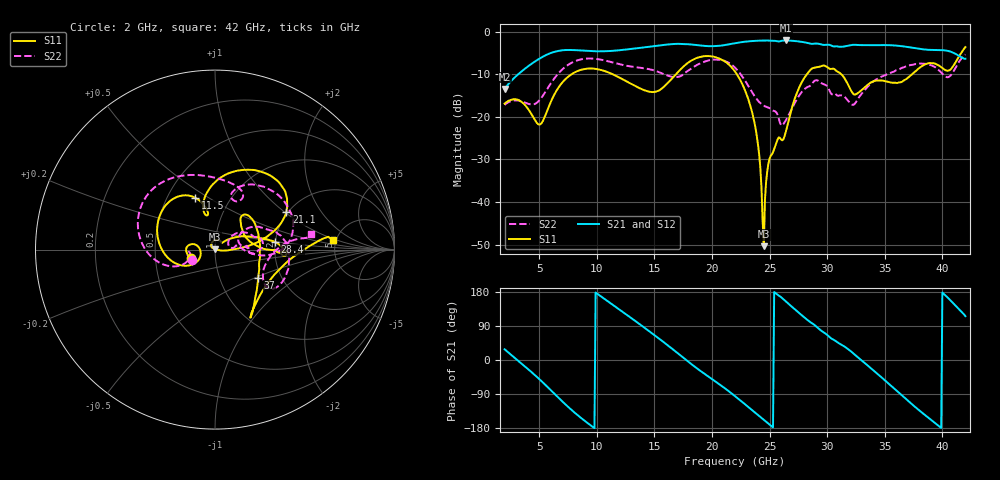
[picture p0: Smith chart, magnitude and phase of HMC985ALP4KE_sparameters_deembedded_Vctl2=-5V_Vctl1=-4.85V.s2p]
!s2p File: Measurements: S11, S21, S12, S22
# GHz S dB R 50.0
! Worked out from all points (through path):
!   401 points, 2 GHz to 42 GHz, reference 50 ohm
!   highest |S21| = -2.06 dB at 26.4 GHz (marker M1); lowest = -13.4 dB at 2 GHz (marker M2)
!   lowest |S11| = -50.4 dB at 24.5 GHz (marker M3), VSWR 1.01, Z = 49.8 + j0.261 ohm
!   |S11| at or under -10 dB: start of sweep to 7.809 GHz; 22.16 GHz to 28.24 GHz (6.081 GHz wide, 24.1 % of centre); 31.22 GHz to 37.36 GHz (6.143 GHz wide, 17.9 % of centre)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
!   |S22| runs from -22.0 to -5.4 dB; largest |S21 - S12| = 0.00096
!   S11 on the Smith chart (normalised r, x): 2 GHz: 0.76, -0.07; 11.5 GHz: 0.68, +0.44; 21.1 GHz: 1.96, +1.02; 28.4 GHz: 1.99, +0.19; 37 GHz: 1.52, -0.52; 42 GHz: 4.71, +0.87
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2  -16.88 -161.7  -13.43 28.3  -13.44 28.3  -17.18 -155.6
5  -21.81 -172.3  -6.37 -50.1  -6.38 -50.1  -16.18 -159.7
6.3  -14.84 -150.2  -4.76 -88.3  -4.76 -88.3  -11.03 -161.5
8.7  -8.91 150.4  -4.44 -154.5  -4.44 -154.5  -6.47 151.4
11.5  -10.16 111.2  -4.47 143.2  -4.48 143.3  -7.31 105.2
13.6  -13.11 101.2  -3.86 97.3  -3.86 97.3  -8.41 75.8
15.4  -13.82 105.8  -3.26 56.6  -3.26 56.6  -9.50 62.2
17.9  -7.34 80.4  -2.95 -3.3  -2.95 -3.3  -9.21 72.2
21.1  -6.97 27.7  -3.15 -74.2  -3.15 -74.1  -6.87 16.3
22  -9.35 17.2  -2.71 -95.3  -2.72 -95.3  -8.45 0.8
23.6  -20.23 0.0  -2.18 -135.0  -2.18 -135.0  -14.71 -4.2
24.5  -50.37 120.1  -2.08 -157.7  -2.08 -157.6  -17.38 8.1
25  -29.80 133.4  -2.11 -170.4  -2.11 -170.3  -17.96 10.8
26.4  -23.62 42.0  -2.06 154.9  -2.06 155.0  -20.87 33.2
28.4  -9.44 7.3  -2.72 103.0  -2.72 103.1  -12.87 18.7
28.7  -8.62 2.3  -2.86 96.8  -2.86 96.8  -12.19 16.7
30.7  -8.96 -2.7  -3.44 50.9  -3.45 50.9  -14.56 2.7
32.5  -14.69 31.8  -3.09 11.3  -3.10 11.3  -16.56 27.7
35.4  -11.83 19.4  -3.17 -64.3  -3.17 -64.2  -9.82 19.6
37  -10.85 -33.1  -3.60 -107.3  -3.60 -107.3  -8.02 5.3
39.8  -8.13 -57.1  -4.31 -176.7  -4.31 -176.7  -9.30 -35.2
42  -3.62 4.5  -6.35 115.7  -6.35 115.7  -5.36 9.0
